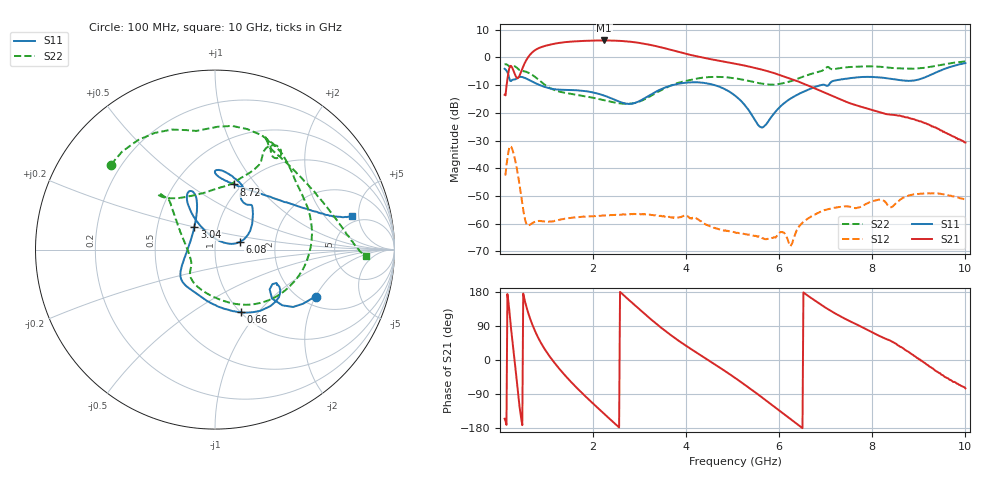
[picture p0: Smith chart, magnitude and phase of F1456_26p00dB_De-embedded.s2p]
! Integrated Device Technology
! Corporate Headquarters
! 6024 Silver Creek Valley Road
! San Jose, CA 95138  USA
! Phone:  1-408-284-8200
! Toll Free:  1-800-223-1366
! Webpage:  http://www.idt.com/
! Timing and RF Division
! 515 Groton Road, Suite 102
! Westford, MA 01886-6024
! Device:  F1456
! Description: 6-bit 0.5 dB Transmit Variable Gain Amplifier
! Frequency:  2100.0 -  2950.00 MHz
! Package:  6x6 mm Thin QFN Plastic Package: 28 pin
! State:  52
! Atten State:  26.0 dB
! Voltage:  +5.00 Volts
! Current:  216.966 mA
! Data:  The device was measured on a the F1455 evaluation board which has
!  individual transmission lines to the RF pins.  Data was collected
!  using a calibrated network analyzer.  The evaluation board was
!  de-embedded using a TRL calibration technique.
!  The reference plane is the edge of the package pin.
!  Pin  1 = CSb
!  Pin  2 = DATA
!  Pin  3 = CLK
!  Pin  4 = RSET
!  Pin  5 = GND
!  Pin  6 = RFIN  = Port 1
!  Pin  7 = GND
!  Pin  8 = NC
!  Pin  9 = NC
!  Pin 10 = NC
!  Pin 11 = NC
!  Pin 12 = NC
!  Pin 13 = NC
!  Pin 14 = /STBY
!  Pin 15 = GND
!  Pin 16 = RFOUT  = Port 2
!  Pin 17 = GND
!  Pin 18 = NC
!  Pin 19 = NC
!  Pin 20 = NC
!  Pin 21 = GND
!  Pin 22 = NC
!  Pin 23 = GND
!  Pin 24 = NC
!  Pin 25 = NC
!  Pin 26 = NC
!  Pin 27 = GND
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# GHz S dB R 50
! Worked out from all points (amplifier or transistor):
!   496 points, 100 MHz to 10 GHz, reference 50 ohm
!   highest |S21| = 6.1 dB at 2.24 GHz (marker M1)
!   |S21| within 3 dB of that: 803.8 MHz to 3.584 GHz (2.78 GHz wide, 127 % of centre)
!   unconditionally stable (mu >= 1): start of sweep to end of sweep
!   at 1.74 GHz: K = 171.85, MAG = 6.4 dB, |S12| = -57.5 dB
!   at 5.06 GHz: K = 750.82, MAG = -1.3 dB, |S12| = -63.2 dB
!   at 10 GHz: K = 692.15, MAG = -21.1 dB, |S12| = -51.3 dB
!   S11 on the Smith chart (normalised r, x): 100 MHz: 2.37, -2.03; 660 MHz: 1.00, -0.82; 3.04 GHz: 0.77, +0.20; 6.08 GHz: 1.31, +0.11; 8.72 GHz: 0.92, +0.78; 10 GHz: 4.17, +4.12
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0.1  -4.12 -24.9  -13.51 -155.0  -42.32 50.0  -2.52 140.8
0.24  -8.55 -31.0  -3.10 81.4  -32.21 -77.1  -3.44 94.5
0.32  -7.97 -29.2  -6.04 -7.1  -36.57 -155.2  -3.25 67.9
0.42  -7.05 -36.7  -6.61 -122.0  -45.83 138.7  -4.58 40.8
0.54  -7.45 -53.5  -1.82 153.6  -58.52 124.5  -5.10 15.2
0.66  -8.46 -67.7  1.21 105.0  -60.20 142.9  -5.98 -12.5
0.84  -9.89 -86.0  3.38 54.3  -58.99 115.9  -8.20 -50.0
1.14  -11.43 -110.6  4.81 -2.4  -59.16 82.3  -11.60 -92.0
1.46  -11.76 -127.8  5.58 -49.0  -58.04 60.5  -12.99 -118.6
1.76  -12.04 -138.9  5.90 -86.8  -57.53 44.4  -13.81 -132.2
2.24  -13.80 -154.5  6.09 -142.1  -57.07 26.1  -15.48 -143.0
2.62  -16.32 180.0  5.89 175.3  -56.70 11.6  -16.70 -156.7
3.04  -15.41 132.7  5.08 128.9  -56.60 -5.4  -15.64 171.1
3.4  -11.98 113.5  3.85 91.5  -57.10 -21.8  -12.44 148.0
4.1  -9.01 112.7  0.84 29.4  -58.01 -54.1  -8.11 133.3
5.06  -13.90 122.9  -2.32 -47.9  -63.23 -104.9  -7.59 135.1
5.62  -25.30 66.6  -4.40 -97.7  -65.01 -160.2  -9.48 119.3
6.08  -16.90 17.0  -6.77 -140.8  -63.17 161.4  -9.34 87.6
6.7  -11.14 40.6  -10.74 162.2  -57.28 148.0  -5.91 63.6
8.36  -7.64 88.7  -20.61 52.6  -53.85 62.3  -3.77 62.5
8.72  -8.45 73.8  -21.62 25.5  -50.26 67.1  -4.06 50.3
10  -2.09 13.9  -30.74 -74.6  -51.31 -25.4  -1.47 -2.6
